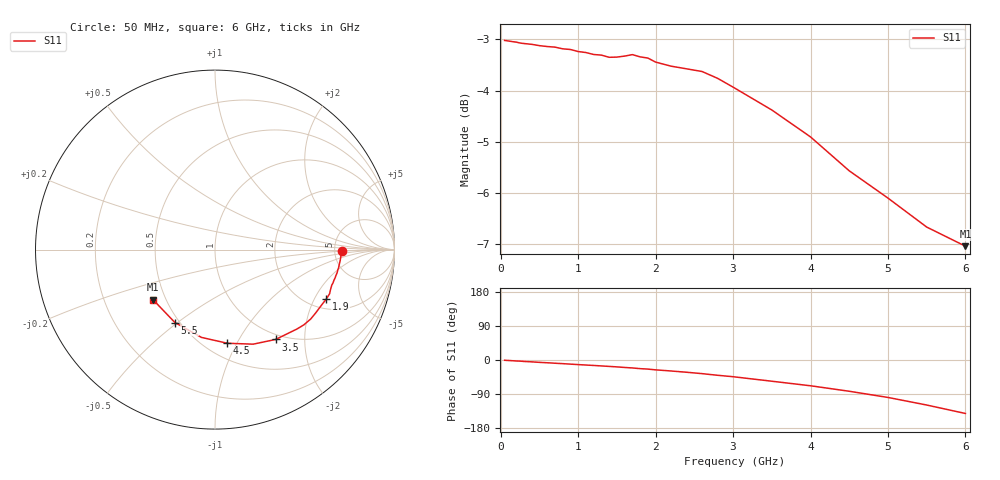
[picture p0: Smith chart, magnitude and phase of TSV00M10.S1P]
! SIEMENS Small Signal Semiconductors
! BAT14-03W
! Si Schottky Diode in SOD323
! IF = 0.1 mA
! S-Parameters:  November  1995
# GHz  S  MA  R  50
!  f  S11
! GHz  MAG  ANG
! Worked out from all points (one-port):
!   34 points, 50 MHz to 6 GHz, reference 50 ohm
!   lowest |S11| = -7.1 dB at 6 GHz (marker M1), VSWR 2.60, Z = 21.3 - j14.8 ohm
!   |S11| at or under -10 dB: nowhere
!   S11 on the Smith chart (normalised r, x): 50 MHz: 5.81, -0.20; 1.9 GHz: 2.44, -2.50; 3.5 GHz: 0.92, -1.45; 4.5 GHz: 0.63, -0.92; 5.5 GHz: 0.47, -0.49; 6 GHz: 0.43, -0.30
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0.05  0.7064 -0.7
0.2  0.7038 -2.6
0.25  0.7023 -3.0
0.3  0.7015 -3.8
0.5  0.6982 -6.2
0.7  0.6958 -8.5
0.8  0.6932 -9.6
1.1  0.6874 -13.3
1.2  0.6844 -14.4
1.3  0.6834 -15.7
1.4  0.6801 -16.9
1.5  0.6804 -18.2
1.6  0.6819 -19.7
1.7  0.6842 -21.0
1.8  0.6807 -22.8
1.9  0.6789 -24.0
2  0.6727 -26.0
2.2  0.6666 -29.0
2.4  0.6626 -32.3
2.6  0.6586 -36.0
2.8  0.6485 -40.3
3  0.6358 -44.1
3.5  0.6038 -56.0
4  0.5682 -68.0
4.5  0.5263 -82.5
5  0.4949 -98.8
5.5  0.4636 -118.8
6  0.444 -141.1
